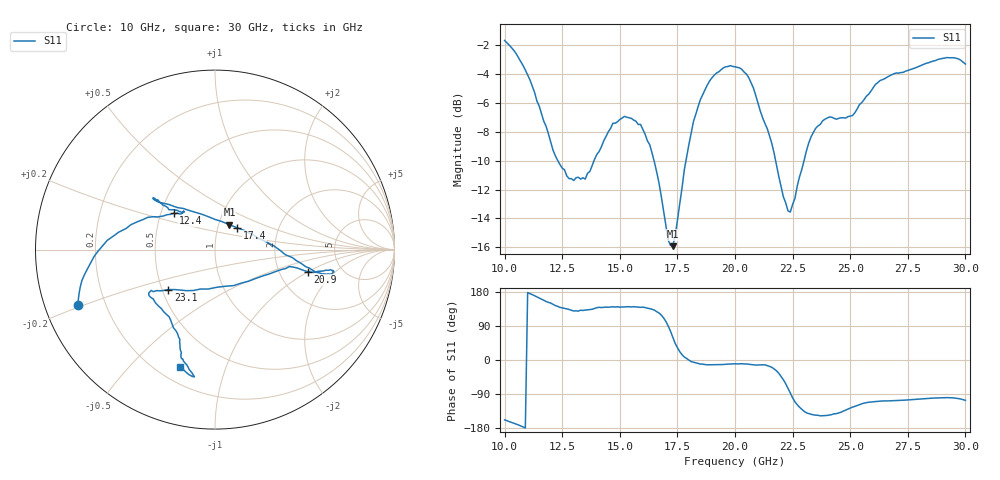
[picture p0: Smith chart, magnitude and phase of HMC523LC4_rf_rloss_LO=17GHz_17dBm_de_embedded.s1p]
!Hittite Microwave Corporation
!20 Alpha Rd
!Chelmsford, MA 01824
!Tel: 978-250-3343
!Fax: 978-250-3373
!Device: HMC523LC4, 10-30 GHz, GaAs MMIC Double-Balanced Mixer
!Misc: RF Return Loss with LO=17GHz at 17 dBm, Room
# MHZ S MA R 50
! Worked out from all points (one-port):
!   201 points, 10 GHz to 30 GHz, reference 50 ohm
!   lowest |S11| = -15.9 dB at 17.3 GHz (marker M1), VSWR 1.38, Z = 56.3 + j16 ohm
!   |S11| at or under -10 dB: 12.31 GHz to 13.88 GHz (1.574 GHz wide, 12 % of centre); 16.49 GHz to 17.87 GHz (1.385 GHz wide, 8.06 % of centre); 21.76 GHz to 23 GHz (1.233 GHz wide, 5.51 % of centre)
!   S11 on the Smith chart (normalised r, x): 10 GHz: 0.10, -0.19; 12.4 GHz: 0.58, +0.26; 17.4 GHz: 1.24, +0.31; 20.9 GHz: 2.89, -0.99; 23.1 GHz: 0.54, -0.27; 30 GHz: 0.29, -0.71
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10000  0.824 -158.0
10600  0.719 -171.4
11300  0.545 169.7
12400  0.307 138.8
12500  0.298 137.7
13500  0.273 131.9
15000  0.439 139.5
15900  0.422 138.9
16300  0.359 135.6
17100  0.168 89.9
17300  0.16 59.8
17400  0.174 44.0
17500  0.196 32.8
18000  0.36 -0.3
18500  0.515 -10.7
19200  0.636 -12.5
20000  0.668 -10.0
20900  0.532 -13.4
21600  0.362 -19.5
22300  0.212 -74.6
22500  0.223 -99.8
23100  0.342 -139.3
24000  0.444 -146.3
25000  0.451 -127.0
26100  0.581 -109.6
27500  0.649 -105.3
29200  0.719 -99.3
30000  0.683 -106.4
